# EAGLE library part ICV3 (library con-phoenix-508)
PHOENIX
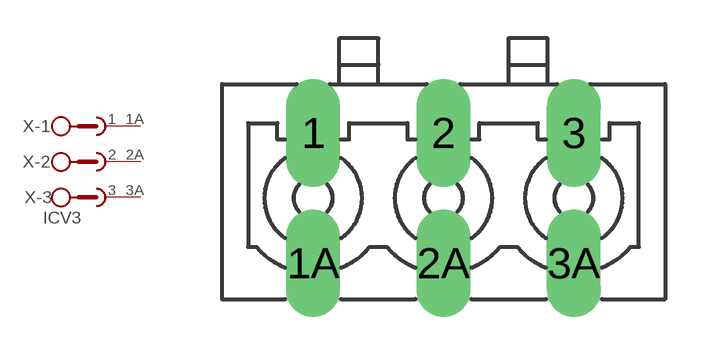
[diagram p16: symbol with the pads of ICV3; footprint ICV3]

Designator prefix X; gates -1=SKB2 -2=SKB2 -3=SKB2V

## ICV3 (OC_FARNELL: unknown; OC_NEWARK: unknown)  [ICV3]
1  -1:1  pas
1A  -1:2  pas
2  -2:1  pas
2A  -2:2  pas
3  -3:1  pas
3A  -3:2  pas

## Footprint ICV3 (pad centres in mm)
PHOENIX
drill 1.397 long: 1 -5.08,2.54; 1A -5.08,-2.54; 2 0,2.54; 2A 0,-2.54; 3 5.08,2.54; 3A 5.08,-2.54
